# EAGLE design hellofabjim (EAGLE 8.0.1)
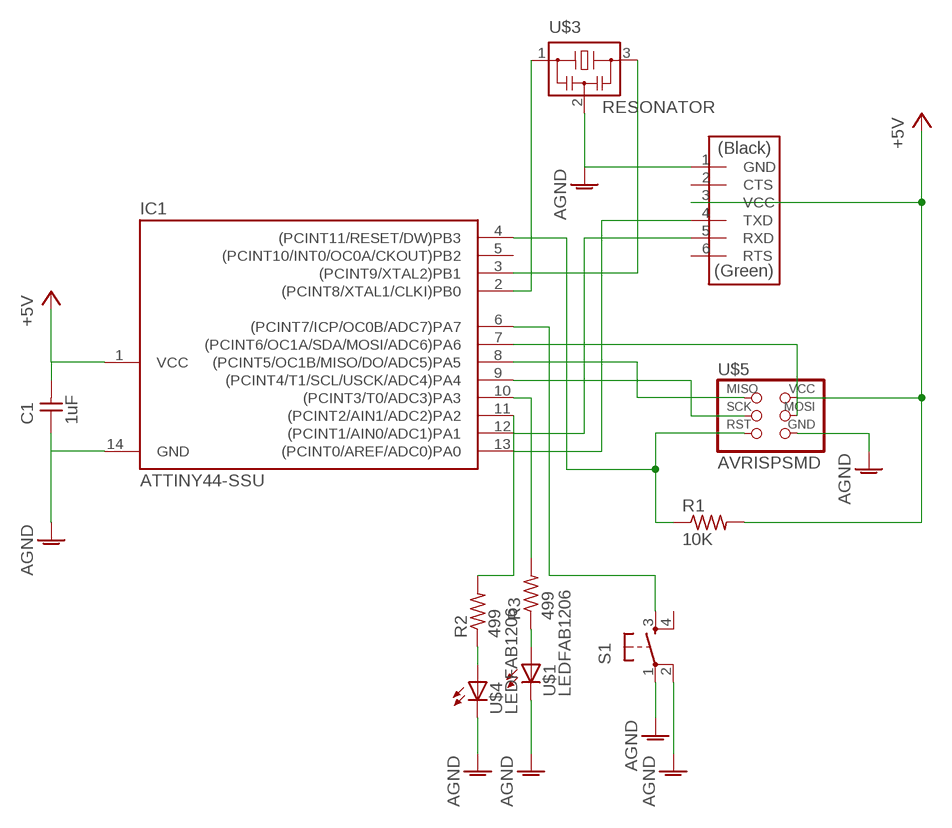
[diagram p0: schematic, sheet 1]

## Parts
C1  1uF  CAP-UNPOLARIZEDFAB  [C1206FAB]
IC1  ATTINY44-SSU  [SOIC14]
R1  10K  RES-US1206FAB  [R1206FAB]
R2  499  RES-US1206FAB  [R1206FAB]
R3  499  RES-US1206FAB  [R1206FAB]
S1  6MM_SWITCH6MM_SWITCH  [6MM_SWITCH]
U$1  LEDFAB1206  [LED1206FAB]
U$2  FTDI-SMD-HEADER  [1X06SMD]
U$3  RESONATOR  [EFOBM]
U$4  LEDFAB1206  [LED1206FAB]
U$5  AVRISPSMD  [2X03SMD]

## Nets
+5V: C1.2 IC1.1(VCC) R1.2 U$2.3(VCC) U$5.2(VCC)
AGND: C1.1 IC1.14(GND) S1.1(P) S1.2(P1) U$1.2(C) U$2.1(GND) U$3.2 U$4.2(C) U$5.6(GND)
N$1: IC1.8((PCINT5/OC1B/MISO/DO/ADC5)PA5) U$5.1(MISO)
N$2: IC1.9((PCINT4/T1/SCL/USCK/ADC4)PA4) U$5.3(SCK)
N$3: IC1.2((PCINT8/XTAL1/CLKI)PB0) U$3.1
N$4: R2.1 U$4.1(A)
N$5: IC1.13((PCINT0/AREF/ADC0)PA0) U$2.4(TXD)
N$6: IC1.12((PCINT1/AIN0/ADC1)PA1) U$2.5(RXD)
N$7: IC1.7((PCINT6/OC1A/SDA/MOSI/ADC6)PA6) U$5.4(MOSI)
N$8: IC1.3((PCINT9/XTAL2)PB1) U$3.3
N$9: IC1.4((PCINT11/RESET/DW)PB3) R1.1 U$5.5(RST)
N$10: IC1.11((PCINT2/AIN1/ADC2)PA2) R2.2
N$11: IC1.10((PCINT3/T0/ADC3)PA3) R3.2
N$12: IC1.6((PCINT7/ICP/OC0B/ADC7)PA7) S1.3(S)
N$13: R3.1 U$1.1(A)
Unconnected: IC1.5((PCINT10/INT0/OC0A/CKOUT)PB2) S1.4(S1) U$2.2(CTS) U$2.6(RTS)

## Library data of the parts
C1 = fab:CAP-UNPOLARIZED
IC1 = fab:ATTINY44
R1-R3 = fab:RES-US: Resistor (US Symbol)
S1 = fab:6MM_SWITCH: OMRON SWITCH
U$1 U$4 = fab:LED: LED
U$2 = fab:FTDI-SMD-HEADER
U$3 = fab:RESONATOR
U$5 = fab:AVRISP

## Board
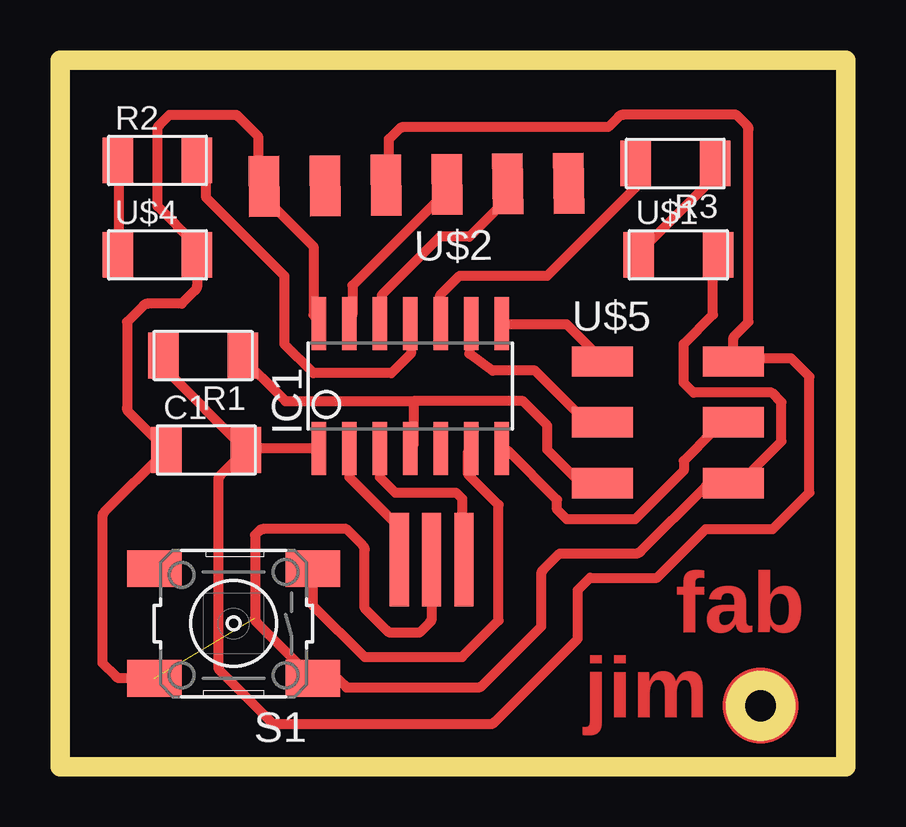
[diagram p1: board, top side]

Size 32.77 x 29.46 mm. Coordinates in mm from the lower left corner, seen from the top.
Outline: 0,0 32.75,0 32.75,29.39 0,29.39 0,0
Outline: 0,0 32.77,0 32.77,29.46 0,29.46 0,0
Outline: circle at 29.21,2.54 radius 1.05
Copper layers (1*16): Top 0.035mm / dielectric 1.5mm / Bottom 0.035mm
Design rules "default *": minimum track width 16mil, minimum drill 24mil, track to track 16mil, track to pad 16mil, pad to pad 16mil, via to via 16mil, smd to smd 0mil, copper to edge 40mil, drill to drill 8mil, minimum pad ring 10mil, minimum via ring 8mil, stop-mask expansion 4mil, vias tented up to drill 0mil, thermal gap 10mil

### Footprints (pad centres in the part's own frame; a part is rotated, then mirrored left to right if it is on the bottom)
C1206FAB = smd 1.27 x 1.905: 1 -1.651,0; 2 1.651,0
SOIC14 = smd 0.61 x 2.21: 1 -3.81,-2.603; 2 -2.54,-2.603; 3 -1.27,-2.603; 4 0,-2.603; 5 1.27,-2.603; 6 2.54,-2.603; 7 3.81,-2.603; 8 3.81,2.603; 9 2.54,2.603; 10 1.27,2.603; 11 0,2.603; 12 -1.27,2.603; 13 -2.54,2.603; 14 -3.81,2.603
R1206FAB = smd 1.27 x 1.905: 1 -1.651,0; 2 1.651,0
6MM_SWITCH = smd 2.286 x 1.524: 1 -3.302,2.286; 2 3.302,2.286; 3 -3.302,-2.286; 4 3.302,-2.286
LED1206FAB = smd 1.27 x 1.905: 1 -1.651,0; 2 1.651,0
1X06SMD = smd 2.54 x 1.27: 1 0,6.35; 2 0,3.81; 3 0,1.27; 4 0,-1.27; 5 0,-3.81; 6 0,-6.35
EFOBM = smd 0.8 x 3.9: 1 -1.35,0; 2 0,0; 3 1.35,0
2X03SMD = smd 2.54 x 1.27: 1 -2.54,2.54; 2 2.92,2.54; 3 -2.54,0; 4 2.92,0; 5 -2.54,-2.54; 6 2.92,-2.54

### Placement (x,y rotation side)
C1  6.1,13.21 0 top
IC1  14.61,15.88 0 top
R1  5.97,17.14 180 top
R2  4.06,25.27 0 top
R3  25.65,25.15 180 top
S1  7.24,5.97 180 top
U$1  25.78,21.34 0 top
U$2  14.86,24.26 90.6 top
U$3  15.49,8.64 0 top
U$4  4.06,21.34 0 top
U$5  25.15,14.35 0 top

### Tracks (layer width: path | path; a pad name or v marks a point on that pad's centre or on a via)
+5V
  Top 0.406: IC1.1 7.94,13.27 C1.2 | R1.2 4.32,16.64 C1.2 | 7.62,13.08 C1.2 | C1.2 6.68,12.14 arc45 6.6,11.96 6.6,4.17 arc45 6.68,3.99 8.89,1.78 17.93,1.78 arc45 18.11,1.85 21.59,5.33 21.59,7.37 22.1,7.87 24.89,7.87 26.92,9.91 29.72,9.91 31.24,11.43 31.24,16.26 30.48,17.02 28.96,17.02 28.7,16.76 28.19,16.76 U$5.2 28.07,17.8 arc-45 28.14,17.98 28.7,18.54 28.7,26.57 arc45 28.63,26.74 28.19,27.18 23.47,27.18 arc45 23.29,27.1 22.86,26.67 14.33,26.67 arc45 14.15,26.6 13.72,26.16 13.72,24.48 | 13.72,24.48 arc-45 13.64,24.3 U$2.3 arc-45 13.66,24.42 13.72,24.48
AGND  (1 unrouted)
  Top 0.406: IC1.14 10.57,18.85 10.57,21.69 8.13,24.13 U$2.1 | U$1.2 27.23,21.29 27.23,18.85 26.01,17.63 26.01,16 26.42,15.6 29.67,15.6 30.07,15.19 30.07,13.56 28.45,11.94 U$5.6 28.01,11.76 arc-45 27.83,11.68 26.92,11.68 24.2,8.96 arc-45 24.02,8.89 20.83,8.89 20.14,8.2 arc45 20.07,8.02 20.07,5.84 17.6,3.38 arc-45 17.42,3.3 11.94,3.3 11.63,3.61 arc45 11.45,3.68 S1.1 8.2,6.02 arc-45 8.13,6.2 8.13,9.65 8.31,9.83 arc-45 8.49,9.91 11.94,9.91 12.63,9.22 arc-45 12.7,9.04 12.7,6.6 13.64,5.66 arc45 13.82,5.59 14.99,5.59 15.42,6.02 arc45 15.49,6.2 U$3.2 | 8.13,24.68 arc45 8.2,24.5 U$2.1 | U$2.1 8.33,24.37 arc-45 8.26,24.55 8.26,26.29 7.44,27.1 arc45 7.26,27.18 4.57,27.18 4.14,26.74 arc45 4.06,26.57 4.06,23.37 5.64,21.79 arc-45 5.71,21.61 U$4.2 5.71,20.04 arc-45 5.64,19.86 5.08,19.3 3.66,19.3 arc45 3.48,19.23 2.79,18.54 2.79,14.96 arc45 2.87,14.79 C1.1 1.85,10.62 arc45 1.78,10.44 1.78,4.32 2.34,3.76 arc45 2.52,3.68 S1.2
N$1
  Top 0.406: IC1.8 18.69,18.44 21.13,18.44 22.35,17.22 U$5.1
N$2
  Top 0.406: IC1.9 17.07,18.44 17.07,17.22 18.03,16.51 19.81,16.51 21.97,14.35 U$5.3 22.35,14.38
N$3
  Top 0.406: 12.06,12.32 IC1.2 12.06,12.06 14.22,9.91 14.22,8.72 U$3.1
N$4
  Top 0.406: U$4.1 2.44,21.69 2.44,24.94 R2.1
N$5
  Top 0.406: IC1.13 12.19,18.85 12.19,20.07 16.26,24.13 U$2.4
N$6
  Top 0.406: IC1.12 13.41,18.85 13.41,19.66 15.85,22.1 17.07,22.1 18.29,23.32 18.29,24.13 U$2.5
N$7
  Top 0.406: IC1.7 18.69,13.16 20.73,11.12 20.73,10.72 21.13,10.31 23.98,10.31 26.01,12.34 26.01,12.75 27.23,13.97 28.04,13.97 U$5.4
N$8
  Top 0.406: 13.41,12.34 13.41,13.16 IC1.3 13.34,12.06 13.97,11.43 16.51,11.43 16.76,11.18 16.76,8.72 U$3.3
N$9
  Top 0.406: U$5.5 21.72,11.81 20.32,13.21 20.32,14.22 19.3,15.24 14.73,15.24 | 14.73,15.24 9.4,15.24 7.37,17.27 R1.1 | 14.73,15.24 14.73,13.4 IC1.4
N$10
  Top 0.406: R2.2 6.1,24.94 6.1,23.72 9.35,20.47 9.35,17.63 10.57,16.41 13.82,16.41 14.63,17.22 14.63,18.44 IC1.11
N$11
  Top 0.406: R3.2 23.98,24.94 23.98,24.13 20.32,20.47 16.66,20.47 15.85,19.66 15.85,18.85 IC1.10
N$12
  Top 0.406: S1.3 10.54,6.73 12.7,4.57 16.76,4.57 18.29,6.1 18.29,10.92 17.02,12.19 17.02,13.14 IC1.6
N$13
  Top 0.406: U$1.1 24.38,21.69 27.64,24.94 R3.1
(copper drawn outside any net)
  shapes: Top circle x1

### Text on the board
Top: fab | jim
